PROGRAM MAIN
VAR
	change: BOOL:=TRUE;
	IGenerator:I_Generator;
	FBGenerator1: FB_Generator;
	FBGenerator2: FB_GeneratorEX;
	input: BOOL;
	tCycletime: TIME:=t#3S;
	sVendor: STRING;
	
END_VAR

IF change THEN
	IGenerator:=FBGenerator1;
ELSE
	IGenerator:=FBGenerator2;
END_IF
				
input := IGenerator.M_Flash();
sVendor:=IGenerator.P_Vendor;
IGenerator.P_Cycletime:=tCycletime;

END_PROGRAM
